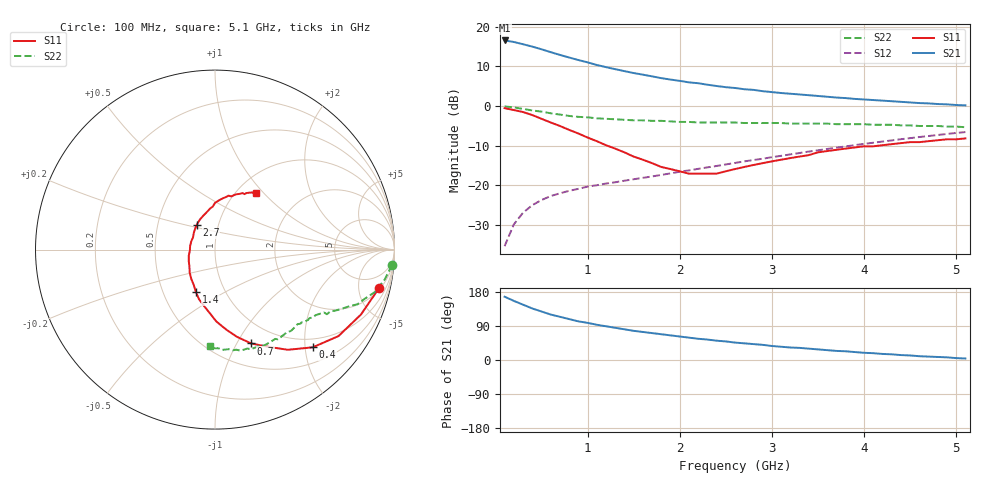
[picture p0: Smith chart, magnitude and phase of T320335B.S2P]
!AT-32033
!S and NOISE PARAMETERS at Vce=5 V  Ic=2mA.  LAST UPDATED 01-05-95
# ghz s ma r 50
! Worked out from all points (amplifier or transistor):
!   51 points, 100 MHz to 5.1 GHz, reference 50 ohm
!   highest |S21| = 16.6 dB at 100 MHz (marker M1)
!   |S21| within 3 dB of that: start of sweep to 606.6 MHz
!   unconditionally stable (mu >= 1): 1.736 GHz to 2.585 GHz; 2.639 GHz to 2.725 GHz
!   at 900 MHz: K = 0.73, MSG = 16.3 dB, |S12| = -20.9 dB
!   at 2.6 GHz: K = 1.00, MSG = 9.5 dB, |S12| = -14.4 dB
!   at 5.1 GHz: K = 0.84, MSG = 3.4 dB, |S12| = -6.6 dB
!   lowest NFmin = 0.52 dB at 500 MHz
!   S11 on the Smith chart (normalised r, x): 100 MHz: 2.25, -8.17; 400 MHz: 0.81, -2.16; 700 MHz: 0.75, -1.15; 1.4 GHz: 0.73, -0.37; 2.7 GHz: 0.79, +0.22; 5.1 GHz: 1.22, +0.91
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0.1  0.94 -13.0  6.73 167.0  0.017 82.0  0.99 -5.0
0.2  0.89 -24.0  6.44 156.0  0.032 76.0  0.96 -10.0
0.3  0.84 -35.0  6.03 146.0  0.045 70.0  0.92 -15.0
0.4  0.77 -45.0  5.63 136.0  0.056 66.0  0.88 -18.0
0.5  0.69 -54.0  5.21 128.0  0.065 62.0  0.85 -21.0
0.6  0.62 -61.0  4.79 120.0  0.073 60.0  0.81 -23.0
0.7  0.56 -69.0  4.42 114.0  0.079 58.0  0.78 -25.0
0.9  0.45 -82.0  3.81 102.0  0.09 56.0  0.73 -28.0
1  0.4 -89.0  3.56 98.0  0.096 55.0  0.72 -30.0
1.1  0.36 -94.0  3.3 93.0  0.1 55.0  0.7 -30.0
1.4  0.26 -114.0  2.76 81.0  0.114 56.0  0.67 -33.0
1.5  0.23 -121.0  2.61 77.0  0.119 56.0  0.66 -35.0
1.8  0.17 -147.0  2.25 68.0  0.135 58.0  0.65 -37.0
2.2  0.14 172.0  1.94 56.0  0.161 59.0  0.62 -42.0
2.4  0.14 151.0  1.79 51.0  0.175 60.0  0.62 -44.0
2.6  0.16 134.0  1.69 46.0  0.191 60.0  0.62 -47.0
2.7  0.17 127.0  1.63 44.0  0.2 60.0  0.61 -49.0
3.1  0.21 104.0  1.46 35.0  0.235 59.0  0.61 -55.0
3.5  0.26 90.0  1.34 28.0  0.276 57.0  0.6 -61.0
4  0.31 76.0  1.21 19.0  0.333 53.0  0.59 -70.0
4.3  0.33 69.0  1.15 15.0  0.368 50.0  0.58 -76.0
5.1  0.39 54.0  1.02 4.0  0.469 41.0  0.54 -93.0
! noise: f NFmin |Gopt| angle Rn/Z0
0.5  0.52  0.79  15  0.42
0.9  0.75  0.65  48  0.3
1.8  1.26  0.33  127  0.11
2.4  1.6  0.39  -166  0.07
